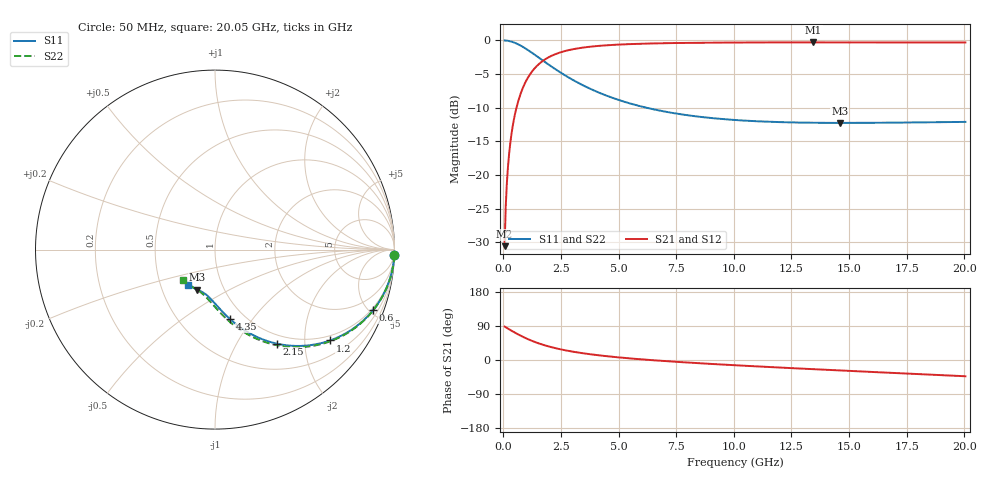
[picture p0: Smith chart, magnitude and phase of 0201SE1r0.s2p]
! AVX Thin Film Operation		Date: August 2001
! Description: Accu-P® Series, Thin Film, SMD, RF Capacitor
! Part Number: 02013J1R0ABW
! 50 MHz  -  20.05 GHz
! Serial Measurements
# mhz S db R 50
!	S11		S21		S12		S22
!	dB	Phase	dB	Phase	dB	Phase	dB	Phase
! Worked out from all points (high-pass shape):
!   401 points, 50 MHz to 20.05 GHz, reference 50 ohm
!   highest |S21| = -0.29 dB at 13.45 GHz (marker M1); lowest = -30.6 dB at 50 MHz (marker M2)
!   |S21| within 3 dB of the highest: 1.617 GHz to end of sweep
!   lowest |S11| = -12.3 dB at 14.6 GHz (marker M3), VSWR 1.64, Z = 37.5 - j17.8 ohm
!   |S11| at or under -10 dB: 6.198 GHz to end of sweep
!   |S22| runs from -12.3 to 0.0 dB; largest |S21 - S12| = 0
!   S11 on the Smith chart (normalised r, x): 50 MHz: 1, -63; 600 MHz: 0.86, -5.25; 1.2 GHz: 0.86, -2.64; 2.15 GHz: 0.86, -1.49; 4.35 GHz: 0.85, -0.78; 20.05 GHz: 0.69, -0.29
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50  -0.00 -1.8  -30.59 88.2  -30.59 88.2  -0.00 -1.8
100  -0.01 -3.6  -24.58 86.3  -24.58 86.3  -0.01 -3.7
200  -0.06 -7.3  -18.61 82.7  -18.61 82.7  -0.06 -7.4
250  -0.09 -9.1  -16.71 80.9  -16.71 80.9  -0.09 -9.2
300  -0.14 -10.8  -15.16 79.1  -15.16 79.1  -0.14 -11.0
450  -0.30 -16.0  -11.81 73.8  -11.81 73.8  -0.30 -16.3
600  -0.51 -21.0  -9.54 68.8  -9.54 68.8  -0.51 -21.4
850  -0.97 -28.8  -6.99 61.0  -6.99 61.0  -0.97 -29.2
1200  -1.75 -38.2  -4.80 51.4  -4.80 51.4  -1.75 -38.8
1600  -2.72 -47.1  -3.33 42.4  -3.33 42.4  -2.72 -47.9
2150  -4.04 -56.6  -2.19 32.8  -2.19 32.8  -4.04 -57.7
2750  -5.35 -64.4  -1.51 24.8  -1.51 24.8  -5.35 -65.8
3400  -6.58 -70.8  -1.09 18.3  -1.09 18.3  -6.58 -72.5
4350  -8.04 -77.8  -0.75 10.9  -0.75 10.9  -8.05 -80.0
5450  -9.33 -84.0  -0.55 4.4  -0.55 4.4  -9.34 -86.7
6750  -10.41 -89.7  -0.43 -1.7  -0.43 -1.7  -10.42 -93.1
10050  -11.83 -101.0  -0.31 -13.8  -0.31 -13.8  -11.86 -105.9
13400  -12.24 -110.4  -0.29 -24.1  -0.29 -24.1  -12.28 -116.8
13450  -12.24 -110.6  -0.29 -24.3  -0.29 -24.3  -12.28 -116.9
14600  -12.26 -113.6  -0.29 -27.6  -0.29 -27.6  -12.30 -120.5
16750  -12.23 -119.2  -0.29 -33.7  -0.29 -33.7  -12.28 -127.0
20050  -12.11 -127.7  -0.30 -42.9  -0.30 -42.9  -12.18 -136.9
